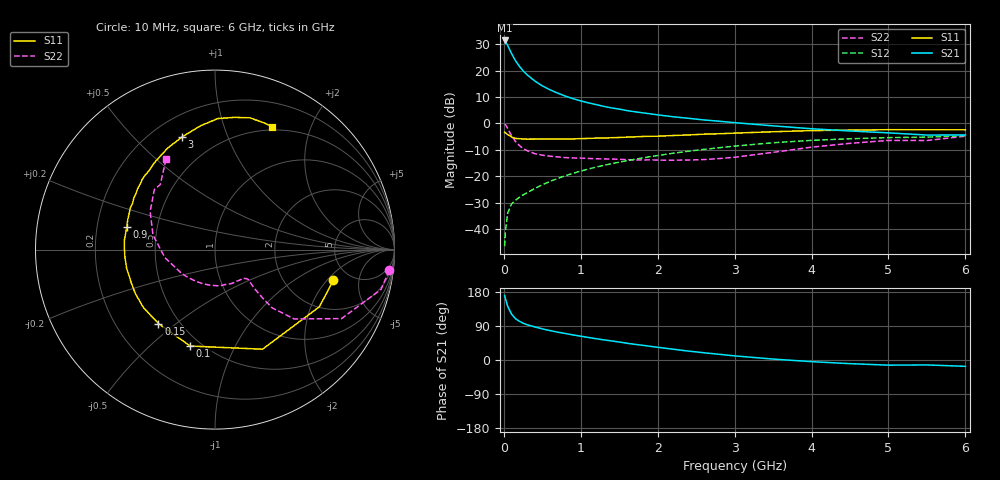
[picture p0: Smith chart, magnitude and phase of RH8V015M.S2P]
! SIEMENS Small Signal Semiconductors
! BFR106
! Si NPN RF Bipolar Junction Transistor in SOT23
! VCE = 8 V  IC = 15 mA
! Common Emitter S-Parameters:  August  1996
# GHz  S  MA  R  50
!  f  S11  S21  S12  S22
! GHz  MAG  ANG  MAG  ANG  MAG  ANG  MAG  ANG
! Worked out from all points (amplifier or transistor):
!   36 points, 10 MHz to 6 GHz, reference 50 ohm
!   highest |S21| = 31.4 dB at 10 MHz (marker M1)
!   |S21| within 3 dB of that: start of sweep to 67.92 MHz
!   unconditionally stable (mu >= 1): 425.9 MHz to 2.054 GHz
!   at 250 MHz: K = 0.81, MSG = 23.5 dB, |S12| = -27.1 dB
!   at 1.4 GHz: K = 1.08, MAG = 8.9 dB, |S12| = -15.3 dB
!   at 6 GHz: K = 0.99, MSG = 0.1 dB, |S12| = -4.6 dB
!   S11 on the Smith chart (normalised r, x): 10 MHz: 3.70, -2.35; 100 MHz: 0.44, -0.68; 150 MHz: 0.38, -0.43; 900 MHz: 0.33, +0.11; 3 GHz: 0.32, +0.70; 6 GHz: 0.46, +1.47
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0.01  0.6814 -14.5  37.36 170.3  0.0047 81.9  0.9786 -6.8
0.02  0.6631 -28.7  36.14 162.5  0.0089 76.7  0.9511 -13.5
0.05  0.6149 -64.5  29.99 141.6  0.02 63.7  0.8031 -28.6
0.1  0.5547 -104.4  21.12 121.3  0.0296 53.1  0.5866 -41.2
0.15  0.5186 -127.4  15.53 109.3  0.0349 51.6  0.4558 -45.5
0.2  0.5132 -140.9  12.23 102.4  0.0396 52.5  0.3828 -45.5
0.25  0.5069 -151.1  9.931 97.1  0.044 54.4  0.3329 -45.0
0.3  0.5018 -158.2  8.385 93.3  0.0482 56.5  0.3052 -44.5
0.4  0.5032 -168.2  6.396 87.4  0.0581 59.5  0.2674 -42.9
0.5  0.5036 -175.4  5.148 82.1  0.0684 62.1  0.2494 -42.0
0.6  0.5054 178.6  4.334 77.7  0.0794 63.4  0.2395 -42.5
0.7  0.5076 173.9  3.745 73.5  0.0903 64.7  0.2316 -44.1
0.9  0.508 165.5  2.942 66.2  0.1133 65.2  0.2207 -47.0
1.1  0.5189 157.2  2.453 59.4  0.1365 64.9  0.2166 -52.9
1.3  0.5265 150.8  2.101 53.1  0.1605 64.0  0.2118 -58.6
1.6  0.5488 141.6  1.75 44.2  0.1963 61.8  0.2056 -70.0
2.2  0.5891 125.3  1.336 28.5  0.2716 55.5  0.2005 -97.5
3  0.6538 106.3  1.033 10.9  0.3706 44.7  0.228 -144.0
3.5  0.6945 96.7  0.898 2.4  0.4293 37.0  0.2825 -170.8
4.5  0.7447 81.6  0.718 -9.6  0.5113 20.5  0.4186 149.7
5.5  0.7572 69.2  0.601 -13.0  0.5486 9.0  0.4735 130.1
6  0.7554 65.0  0.604 -16.7  0.5869 1.2  0.5724 118.5
